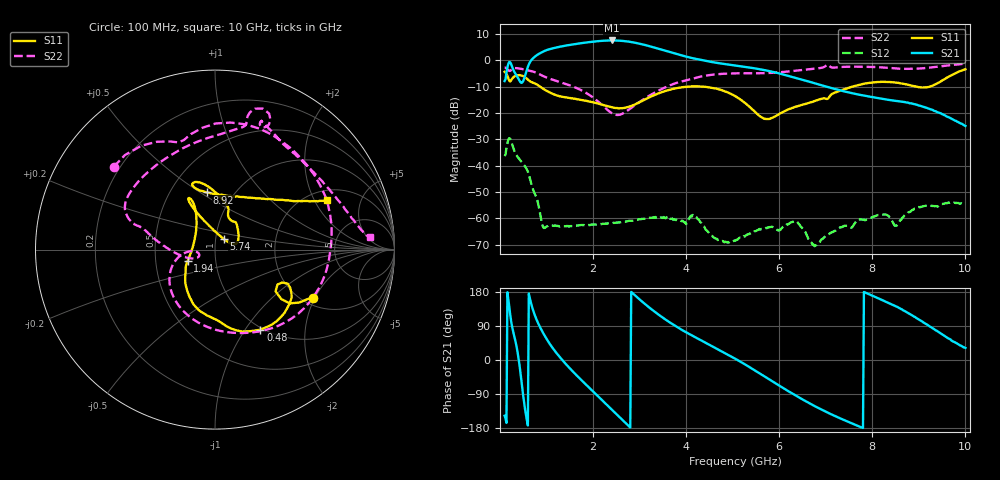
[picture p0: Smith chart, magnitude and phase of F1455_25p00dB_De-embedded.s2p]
! Integrated Device Technology
! Corporate Headquarters
! 6024 Silver Creek Valley Road
! San Jose, CA 95138  USA
! Phone:  1-408-284-8200
! Toll Free:  1-800-223-1366
! Webpage:  http://www.idt.com/
! Timing and RF Division
! 515 Groton Road, Suite 102
! Westford, MA 01886-6024
! Device:  F1455
! Description: 6-bit 0.5 dB Transmit Variable Gain Amplifier
! Frequency:  1400.0 -  2300.00 MHz
! Package:  6x6 mm Thin QFN Plastic Package: 28 pin
! State:  50
! Atten State:  25.0 dB
! Voltage:  +5.00 Volts
! Current:  217.636 mA
! Data:  The device was measured on a the F1455 evaluation board which has
!  individual transmission lines to the RF pins.  Data was collected
!  using a calibrated network analyzer.  The evaluation board was
!  de-embedded using a TRL calibration technique.
!  The reference plane is the edge of the package pin.
!  Pin  1 = CSb
!  Pin  2 = DATA
!  Pin  3 = CLK
!  Pin  4 = RSET
!  Pin  5 = GND
!  Pin  6 = RFIN  = Port 1
!  Pin  7 = GND
!  Pin  8 = NC
!  Pin  9 = NC
!  Pin 10 = NC
!  Pin 11 = NC
!  Pin 12 = NC
!  Pin 13 = NC
!  Pin 14 = /STBY
!  Pin 15 = GND
!  Pin 16 = RFOUT  = Port 2
!  Pin 17 = GND
!  Pin 18 = NC
!  Pin 19 = NC
!  Pin 20 = NC
!  Pin 21 = GND
!  Pin 22 = NC
!  Pin 23 = GND
!  Pin 24 = NC
!  Pin 25 = NC
!  Pin 26 = NC
!  Pin 27 = GND
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# GHz S dB R 50
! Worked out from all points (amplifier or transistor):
!   496 points, 100 MHz to 10 GHz, reference 50 ohm
!   highest |S21| = 7.6 dB at 2.4 GHz (marker M1)
!   |S21| within 3 dB of that: 1.133 GHz to 3.385 GHz (2.252 GHz wide, 99.7 % of centre)
!   unconditionally stable (mu >= 1): start of sweep to end of sweep
!   at 1.74 GHz: K = 283.28, MAG = 7.0 dB, |S12| = -62.6 dB
!   at 5.06 GHz: K = 1075.25, MAG = 0.0 dB, |S12| = -68.5 dB
!   at 10 GHz: K = 626.79, MAG = -16.2 dB, |S12| = -54.4 dB
!   S11 on the Smith chart (normalised r, x): 100 MHz: 2.27, -1.94; 480 MHz: 0.97, -1.18; 1.94 GHz: 0.73, -0.09; 5.74 GHz: 1.09, +0.13; 8.92 GHz: 0.75, +0.53; 10 GHz: 2.45, +2.53
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0.1  -4.30 -26.1  -7.82 -147.2  -36.38 47.6  -2.75 140.7
0.18  -6.74 -36.7  -1.28 160.6  -30.14 -6.6  -3.72 112.5
0.26  -6.97 -25.1  -2.31 88.3  -31.67 -77.2  -3.32 96.0
0.38  -5.62 -42.4  -6.37 19.5  -36.71 -118.4  -2.99 58.1
0.48  -5.81 -60.5  -8.38 -74.5  -38.89 -149.8  -3.26 31.5
0.66  -8.08 -88.0  -0.21 153.7  -46.03 141.6  -3.99 -10.6
0.8  -9.21 -105.8  2.11 102.7  -53.02 112.4  -4.81 -41.7
0.96  -11.12 -123.5  3.63 64.3  -63.64 128.8  -6.18 -71.2
1.34  -13.81 -143.6  5.41 -0.2  -63.02 110.6  -8.49 -121.0
1.76  -15.01 -153.5  6.61 -54.3  -62.55 81.6  -11.44 -156.1
1.94  -15.68 -157.6  7.02 -75.8  -62.58 73.3  -13.35 -167.0
2.4  -17.77 -178.9  7.61 -130.7  -61.82 57.7  -20.01 -171.6
2.82  -17.32 143.1  7.01 179.7  -60.90 47.5  -18.06 -157.1
3.4  -12.54 117.1  4.53 120.4  -59.55 26.5  -11.54 178.3
4.08  -9.92 116.3  1.12 67.7  -59.50 13.7  -7.21 163.0
5.06  -13.61 114.5  -1.92 3.0  -68.52 23.6  -4.89 148.1
5.74  -22.32 51.7  -3.86 -47.5  -63.75 23.1  -4.79 120.0
6.36  -17.56 18.7  -6.63 -94.1  -61.08 -25.7  -3.91 88.7
6.7  -15.81 37.1  -8.35 -117.7  -69.36 -139.8  -3.21 78.6
8.36  -8.17 108.6  -15.02 149.8  -59.34 70.2  -2.82 62.6
8.92  -9.85 98.0  -16.66 113.6  -56.37 92.9  -3.15 40.1
10  -3.33 23.9  -24.89 31.9  -54.42 20.5  -1.27 4.6
